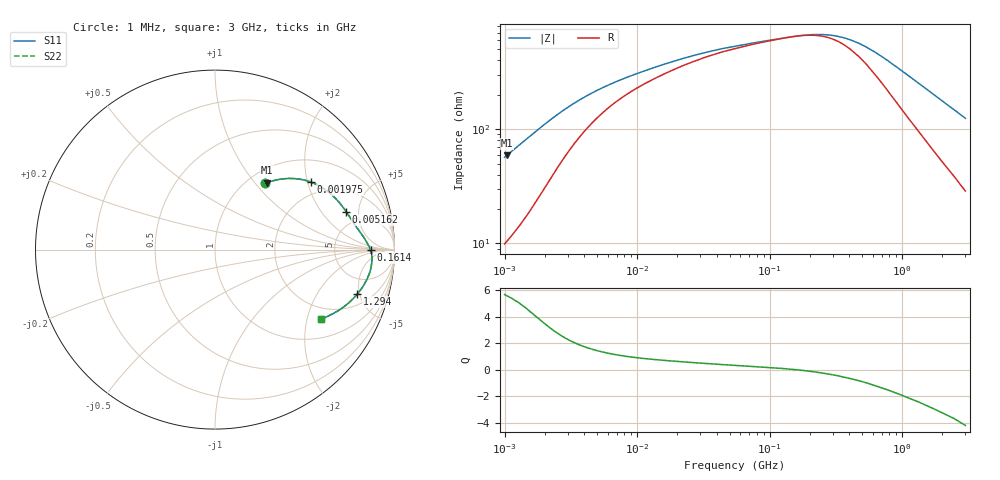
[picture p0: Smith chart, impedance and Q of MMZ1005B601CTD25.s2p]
! S-Parameter Data Generated by TDK Corporation
! Copyright(C) 2025 TDK Corporation.
! All Rights Reserved.
! TDK P/N: MMZ1005B601CTD25 (Chip Bead)
! Property: |Z|=600ohm at 100MHz
! Size(LxWxT): 1x0.5x0.5mm
! Model Type: s2p (Touchstone File Format Version 1.0)
! Frequency: DC=Yes Start=1MHz Stop=3000MHz 202points Log-sweep
! Model Generated on Feb. 6, 2025
! Terms and conditions regarding TDK Simulation Models:
! 1)This simulation model is being provided solely for informational
!  purposes. Please refer to the specifications of the products in
!  terms of detailed characteristics of such products.
! 2)In no event shall TDK Corporation of any of its subsidiaries be
!  liable for any loss or damage arising, directly or indirectly,
!  from any information contained in this simulation model, including,
!  but not limited to loss or damages arising from any inaccuracies,
!  omissions or errors in connection with such information.
! 3)Any and all copyrights on this simulation model are owned by
!  TDK Corporation.  Duplication or redistribution of this simulation
!  model without prior written permission from TDK Corporation
!  is prohibited.
! 4)This simulation model is subject to any modification or change
!  without any prior notice.
! 5)Neither TDK Corporation nor any of its subsidiaries shall make any
!  warranty, express or implied, including but not limited to the
!  correctness, implied warranties of merchantability and fitness for
!  a particular purpose with respect to this simulation models.
! 6)The use of this simulation model shall be deemed to have consented
!  to the terms and conditions hereof.
! Port Assignments:
!  1 ---@@@--- 2
! Applicable Conditions:
!  Temperature = 25 degC
!  DC Bias Current = 0 A
!  Small Signal Operation
# Hz S MA R 50
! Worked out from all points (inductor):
!   201 points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, 1 MHz to 3 GHz, reference 50 ohm
!   read as one part in series: L = 8.8 uH near 1.041 MHz
!   highest Q = 5.56 at 1.041 MHz (marker M1), where L = 8.91 uH
!   self-resonance near 153.9 MHz
!   S11 on the Smith chart (normalised r, x): 1 MHz: 1.20, +1.12; 1.975 MHz: 1.60, +2.09; 5.162 MHz: 3.60, +3.62; 161.4 MHz: 14, -0; 1.294 GHz: 2.99, -4.77; 3 GHz: 1.58, -2.42
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1000000  0.4615 52.9  0.8104 -27.0  0.8104 -27.0  0.4615 52.9
1040844  0.474 52.0  0.8007 -27.8  0.8007 -27.8  0.474 52.0
1433740  0.5712 44.0  0.7099 -34.0  0.7099 -34.0  0.5712 44.0
1682724  0.615 39.6  0.6562 -36.7  0.6562 -36.7  0.615 39.6
1974946  0.6528 35.2  0.5998 -38.9  0.5998 -38.9  0.6528 35.2
2720446  0.7075 27.2  0.492 -41.1  0.492 -41.1  0.7075 27.2
3900413  0.7431 20.2  0.3962 -40.3  0.3962 -40.3  0.7431 20.2
5161903  0.7611 16.1  0.3416 -38.1  0.3416 -38.1  0.7611 16.1
8345207  0.7845 11.2  0.2764 -33.5  0.2764 -33.5  0.7845 11.2
1.461624e7  0.8082 7.6  0.226 -28.3  0.226 -28.3  0.8082 7.6
2.886629e7  0.8318 4.7  0.1841 -21.8  0.1841 -21.8  0.8318 4.7
5.477226e7  0.8468 2.7  0.1594 -14.7  0.1594 -14.7  0.8468 2.7
1.614254e8  0.8672 -0.2  0.1328 1.0  0.1328 1.0  0.8672 -0.2
2.136344e8  0.8718 -1.2  0.1297 8.1  0.1297 8.1  0.8718 -1.2
3.062963e8  0.8759 -2.9  0.1331 19.7  0.1331 19.7  0.8759 -2.9
4.0536e8  0.8766 -4.6  0.1449 29.3  0.1449 29.3  0.8766 -4.6
5.364635e8  0.8746 -6.8  0.1673 38.2  0.1673 38.2  0.8746 -6.8
8.005644e8  0.8635 -10.8  0.2223 46.9  0.2223 46.9  0.8635 -10.8
1.294266e9  0.8311 -17.3  0.3216 50.1  0.3216 50.1  0.8311 -17.3
1.645649e9  0.8055 -21.2  0.3835 49.5  0.3835 49.5  0.8055 -21.2
2.01032e9  0.7781 -24.9  0.4405 48.1  0.4405 48.1  0.7781 -24.9
3e9  0.7044 -33.4  0.5656 43.3  0.5656 43.3  0.7044 -33.4
